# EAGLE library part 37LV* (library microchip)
Serial EPROM 36 K/64 K/128 K
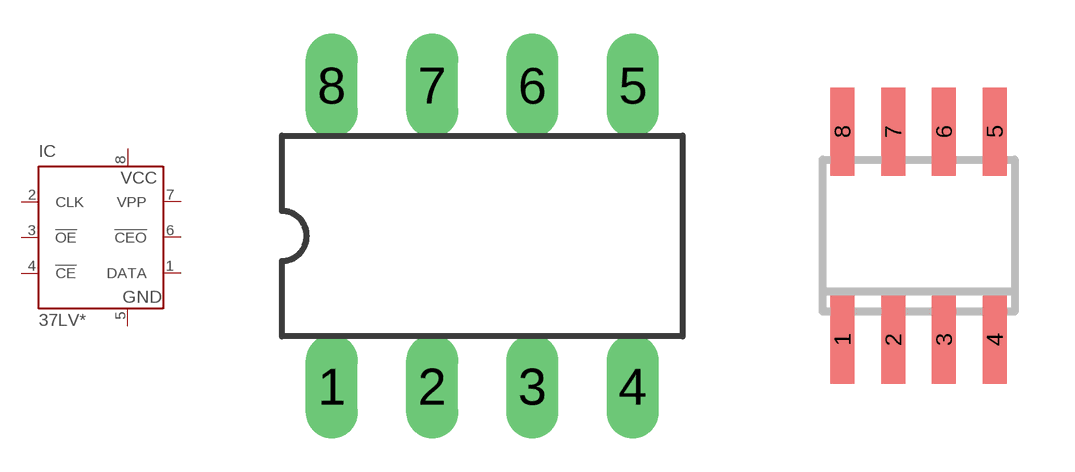
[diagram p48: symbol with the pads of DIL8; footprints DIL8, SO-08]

Designator prefix IC

## 37LV128P (OC_FARNELL: unknown; OC_NEWARK: unknown), 37LV36P (OC_FARNELL: unknown; OC_NEWARK: unknown), 37LV65P (OC_FARNELL: unknown; OC_NEWARK: unknown)  [DIL8]
1  DATA  hiz
2  CLK  in
3  !OE  in
4  !CE  in
5  GND  pwr
6  !CEO  out
7  VPP  in
8  VCC  pwr

## 37LV128SN (OC_FARNELL: unknown; OC_NEWARK: unknown), 37LV36SN (OC_FARNELL: unknown; OC_NEWARK: unknown), 37LV65SN (OC_FARNELL: unknown; OC_NEWARK: unknown)  [SO-08]
Pads as for DIL8

## 37LV128L (OC_FARNELL: unknown; OC_NEWARK: unknown), 37LV36L (OC_FARNELL: unknown; OC_NEWARK: unknown), 37LV65L (OC_FARNELL: unknown; OC_NEWARK: unknown)  [PLCC20S]
2  DATA  hiz
4  CLK  in
6  !OE  in
8  !CE  in
10  GND  pwr
14  !CEO  out
17  VPP  in
20  VCC  pwr

## Footprint DIL8 (pad centres in mm)
Dual In Line package type P
drill 0.813 long: 1 -3.81,-3.81; 2 -1.27,-3.81; 3 1.27,-3.81; 4 3.81,-3.81; 5 3.81,3.81; 6 1.27,3.81; 7 -1.27,3.81; 8 -3.81,3.81

## Footprint SO-08 (pad centres in mm)
Small Outline Narrow Plastic Gull Wing 150-mil body, package type SN
smd 0.6 x 2.2: 1 -1.905,-2.6; 2 -0.635,-2.6; 3 0.635,-2.6; 4 1.905,-2.6; 5 1.905,2.6; 6 0.635,2.6; 7 -0.635,2.6; 8 -1.905,2.6

## Footprint PLCC20S (pad centres in mm)
PLASTIC LEADED CHIP CARRIER square, package type L
smd 0.6 x 2.2: 1 0,4.3; 2 -1.27,4.3; 3 -2.54,4.3; 9 -2.54,-4.3; 10 -1.27,-4.3; 11 0,-4.3; 12 1.27,-4.3; 13 2.54,-4.3; 19 2.54,4.3; 20 1.27,4.3
smd 2.2 x 0.6: 4 -4.3,2.54; 5 -4.3,1.27; 6 -4.3,0; 7 -4.3,-1.27; 8 -4.3,-2.54; 14 4.3,-2.54; 15 4.3,-1.27; 16 4.3,0; 17 4.3,1.27; 18 4.3,2.54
